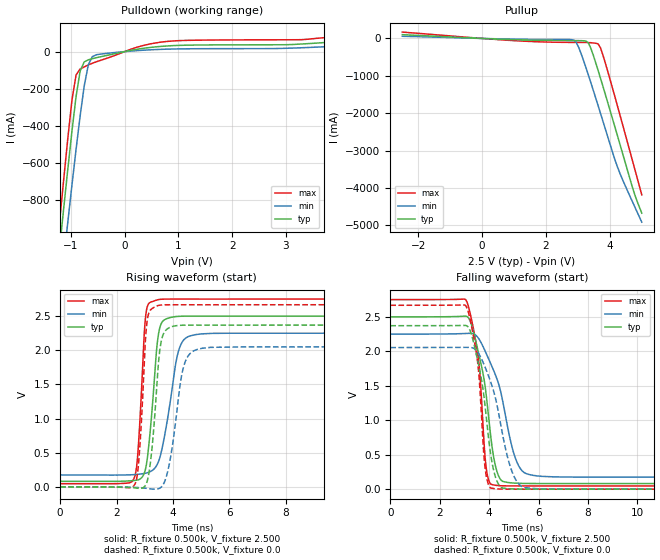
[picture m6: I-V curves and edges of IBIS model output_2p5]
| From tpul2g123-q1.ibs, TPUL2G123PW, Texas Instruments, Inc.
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|   Model output_2p5
[Model] output_2p5
Model_type Output
Polarity   Non-Inverting
Enable   Active-High
Vmeas = 2.5v
Cref = 15pf
C_comp   2.213pF   1.945pF   2.486pF
[Temperature Range]   27.000   0.125k   -40.000
[Voltage Range]   2.500V   2.250V   2.750V
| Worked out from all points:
|   slope of the pulldown table from 0 to 0.375 V, typ, clamps not added: 20.1 ohm
|   slope of the pullup table from 0 to 0.375 V, typ, clamps not added: 27.8 ohm
|   rising waveform, R_fixture 0.500k, V_fixture 2.500: 20-80 % time 290ps typ, 483ps min, 207ps max; typ from 0.082 V to 2.5 V
|   rising waveform, R_fixture 0.500k, V_fixture 0.0: 20-80 % time 272ps typ, 407ps min, 206ps max; typ from 0 V to 2.37 V
|   falling waveform, R_fixture 0.500k, V_fixture 2.500: 20-80 % time 594ps typ, 897ps min, 384ps max; typ from 2.5 V to 0.082 V
|   falling waveform, R_fixture 0.500k, V_fixture 0.0: 20-80 % time 559ps typ, 812ps min, 371ps max; typ from 2.37 V to 0 V
[Pulldown]
|Voltage   I(typ)   I(min)   I(max)
-2.5V     -4.657A    -4.448A    -4.894A
-1.208V   -1.051A    -1.318A    -908mA
-1.132V   -837.6mA   -1.114A    -681.9mA
-1.056V   -628.3mA   -913.3mA   -462.9mA
-980mV    -426.9mA   -716.5mA   -260.1mA
-904mV    -241.4mA   -525.8mA   -125.7mA
-828mV    -104.1mA   -345.3mA   -93.61mA
-676mV    -44.2mA    -70.63mA   -71.71mA
-524mV    -32.55mA   -16.72mA   -54.42mA
768mV     30.01mA    13mA       54.11mA
3.276V    40.72mA    20.58mA    64.18mA
5V        78.97mA    17.86mA    118.9mA
[Pullup]
|Voltage   I(typ)   I(min)   I(max)
-2.5V     101mA      58.69mA    170.1mA
896mV     -30.11mA   -16.83mA   -53mA
2.796V    -57.39mA   -30.41mA   -105.6mA
2.948V    -57.88mA   -106.2mA   -106.5mA
3.252V    -70.51mA   -781.2mA   -108.1mA
3.328V    -119.1mA   -978.6mA   -109.9mA
3.404V    -261.5mA   -1.18A     -114.1mA
3.632V    -853.7mA   -1.796A    -145.4mA
3.708V    -1.066A    -2.004A    -254.1mA
4.24V     -2.606A    -3.44A     -1.81A
4.772V    -4.156A    -4.486A    -3.466A
5V        -4.671A    -4.912A    -4.181A
[Ramp]
| variable   typ   min   max
dV/dt_r   1.423/0.272n   1.232/0.407n   1.601/0.207n
dV/dt_f   1.451/0.595n   1.245/0.897n   1.622/0.384n
R_load = 0.500k
[Rising Waveform]
R_fixture= 0.500k
V_fixture= 2.500
V_fixture_min= 2.250
V_fixture_max= 2.750
|time   V(typ)   V(min)   V(max)
0s        81.54mV    174.6mV    46.56mV
2.595ns   92.25mV    179.1mV    102.9mV
2.766ns   102.9mV    184.6mV    548.6mV
2.981ns   198.3mV    196.1mV    2.229V
3.047ns   299.5mV    201.8mV    2.547V
3.427ns   2.036V     316.5mV    2.736V
3.527ns   2.318V     417.1mV    2.745V
4.231ns   2.497V     2.033V     2.75V
5.043ns   2.5V       2.241V     2.75V
50ns      2.5V       2.25V      2.75V
[Rising Waveform]
R_fixture= 0.500k
V_fixture= 0.0
V_fixture_min= 0.0
V_fixture_max= 0.0
|time   V(typ)   V(min)   V(max)
0s        563.3nV    416.5nV    837.7nV
2.654ns   -14.39mV   -7.281mV   41.25mV
2.815ns   -21.51mV   -10.71mV   525.3mV
3.08ns    74.57mV    -22.02mV   2.414V
3.263ns   588mV      -31.92mV   2.612V
3.543ns   2.029V     -16.01mV   2.661V
3.89ns    2.335V     372.7mV    2.666V
4.391ns   2.367V     1.779V     2.666V
5.041ns   2.368V     2.03V      2.666V
50ns      2.371V     2.054V     2.668V
[Falling Waveform]
R_fixture= 0.500k
V_fixture= 2.500
V_fixture_min= 2.250
V_fixture_max= 2.750
|time   V(typ)   V(min)   V(max)
0s        2.5V       2.25V      2.75V
3.062ns   2.509V     2.259V     2.742V
3.565ns   1.982V     2.19V      1.892V
3.815ns   1.544V     2.021V     557.3mV
3.908ns   1.279V     1.947V     243.1mV
4.247ns   348.7mV    1.664V     56.94mV
4.503ns   124.2mV    1.355V     49.36mV
5.121ns   86.4mV     394.3mV    47.09mV
6.141ns   81.75mV    185.6mV    46.6mV
50ns      81.54mV    174.6mV    46.56mV
[Falling Waveform]
R_fixture= 0.500k
V_fixture= 0.0
V_fixture_min= 0.0
V_fixture_max= 0.0
|time   V(typ)   V(min)   V(max)
0s        2.371V     2.054V     2.668V
3.058ns   2.374V     2.057V     2.657V
3.535ns   1.867V     1.99V      1.833V
3.778ns   1.38V      1.82V      536.7mV
3.868ns   1.098V     1.741V     223.3mV
4.194ns   255mV      1.405V     8.776mV
4.454ns   35.15mV    965mV      1.821mV
4.924ns   4.224mV    255.1mV    204.4uV
5.558ns   438.6uV    17.63mV    65.98uV
50ns      863.1nV    4.099uV    156.3nV
